|   18XX
[IBIS ver]   4.1
[File name]   18xx.ibs
[File Rev]   1.0
[Date]   Apr 18, 2014
[Source]   Data created at Texas Instruments India
[Disclaimer]   This information is for modeling purpose only, and is not
   guaranteed. The information is subject to change without
   notice.
[Copyright] Texas Instruments
|   Component 18XX
[Component]   18XX
[Manufacturer]   Texas Instruments.
[Package]
| variable   typ   min   max
R_pkg   0.35113   0.0058816   1.09261
L_pkg   8.95381e-10   1.49981e-11   2.78616e-09
C_pkg   2.63203e-13   2.01059e-13   3.9667e-13
[Pin]  signal_name   model_name   R_pin   L_pin   C_pin
A1   VSS_WL   NC   0   0   0
A2   RF_IN1_A_WL   NC   0   0   0
A3   VDD_OUT_VCO_WL   NC   0   0   0
A4   RF_IN2_A_WL   NC   0   0   0
A5   VSS_ANT_BG_WL   NC   0   0   0
A6   VDD_IN_PA_BG_WL   NC   0   0   0
A7   RF_IO1_BG_WL   NC   0   0   0
A8   VSS_RF_BT   NC   0   0   0
A9   RF_IO_BT   NC   0   0   0
A10  VSS_DCO_BT   NC   0   0   0
A11  VPP   NC   0   0   0
B1   RF_OUT_A_WL   NC   0   0   0
B2   VSS_PA_A_WL   NC   0   0   0
B3   VSS_VCO_WL   NC   0   0   0
B4   DEPOP   NC   0   0   0
B5   VDD_OUT_RF_WL   NC   0   0   0
B6   VSS_RF_WL   NC   0   0   0
B7   VSS_RF_WL   NC   0   0   0
B8   VDD_OUT_PPA_IF_BT   NC   0   0   0
B9   VDD_OUT_RF_BT   NC   0   0   0
B10  VDD_OUT_DCO_BT   NC   0   0   0
B11  FUNC2_BT   BQ18PROGHHVHYFBPB_IUANV_6LM   0.107178   2.73303e-10   2.19292e-13
C1   VSS_ANT_WL   NC   0   0   0
C2   VDD_IN_PA_WL   NC   0   0   0
C3   LDO_IN_WL   NC   0   0   0
C4   VDD_OUT_ANA_WL   NC   0   0   0
C5   VSS_ANA_WL   NC   0   0   0
C6   PDET_IN_FEM_TESTM_WL   OQ18120COMPFZPD_IUAJH_6LM   1.09261   2.78616e-09   3.9667e-13
C7   PABIAS_OUT_FEM_TESTP_WL   NC   0   0   0
C8   VDD_OUT_PA_BT   NC   0   0   0
C9   LDO_IN_PA_BT   NC   0   0   0
C10  LDO_IN_BT   NC   0   0   0
C11  VIO_IN   NC   0   0   0
D1   RF_IO2_BG_WL   NC   0   0   0
D2   VSS_PA_BG_WL   NC   0   0   0
D3   DC2DC_REQ_OUT   BQ18PROGHHVHYFBPB_IUANH_6LM   0.419876   1.07068e-09   2.75578e-13
D4   VSS_CLK   NC   0   0   0
D5   VSS   NC   0   0   0
D6   RF_SW_WL   NC   0   0   0
D7   VDD_DIG   NC   0   0   0
D8   SDIO_CMD_WL   BQ18PROGHHVHYFBPB_IUANH_6LM   0.529399   1.34997e-09   2.95292e-13
D9   VSS   NC   0   0   0
D10  SDIO_D3_WL   BQ18PROGHHVHYFBPB_IUANH_6LM   0.225237   5.74355e-10   2.40543e-13
D11  SDIO_D2_WL   BQ18PROGHHVHYFBPB_IUANH_6LM   0.0531736   1.35593e-10   2.09571e-13
E1   WL_EN   IQ18HHVHYSINK_IUAJH_6LM   0.0467988   1.19337e-10   2.08424e-13
E2   BT_EN   IQ18HHVHYSINK_IUAJH_6LM   0.20561   5.24306e-10   2.3701e-13
E3   IRQ_WL   BQ18PROGHHVHYFBPB_IUANH_6LM   0.357414   9.11405e-10   2.64334e-13
E4   CLK_IN_P   NC   0   0   0
E5   CLK_IN_M   NC   0   0   0
E6   RF_SW_BT   NC   0   0   0
E7   HCI_RX_BT   BQ18PROGHHVHYFBPB_IUANH_6LM   0.614975   1.56819e-09   3.10695e-13
E8   FUNC1_BT   BQ18PROGHHVHYFBPB_IUANV_6LM   0.491606   1.2536e-09   2.88489e-13
E9   SDIO_D1_WL   BQ18PROGHHVHYFBPB_IUANH_6LM   0.34553   8.81102e-10   2.62195e-13
E10  SDIO_D0_WL   BQ18PROGHHVHYFBPB_IUANH_6LM   0.210326   5.36332e-10   2.37859e-13
E11  SDIO_CLK_WL   BQ18PROGHHVHYFBPB_IUANH_6LM   0.0593028   1.51222e-10   2.10675e-13
F1   TX_SW_FEM_WL   BQ18SMART1HYFBPB_IUAJH_6LM   0.0551497   1.40632e-10   2.09927e-13
F2   PA_EN_FEM_WL   BQ18SMART1HYFBPB_IUAJH_6LM   0.20123   5.13136e-10   2.36221e-13
F3   RX_SW_FEM_WL   BQ18SMART1HYFBPB_IUAJH_6LM   0.351615   8.96619e-10   2.63291e-13
F4   RF_SW_1P8V_WL   BQ18SMART1HYFBPB_IUAJH_6LM   0.49319   1.25763e-09   2.88774e-13
F5   VDD_DIG   NC   0   0   0
F6   HCI_CTS_BT   BQ18PROGHHVHYFBPB_IUANH_6LM   0.751778   1.91703e-09   3.3532e-13
F7   HCI_TX_BT   BQ18PROGHHVHYFBPB_IUANH_6LM   0.621592   1.58506e-09   3.11886e-13
F8   I2S_FSYNC_FM   BQ18PROGHHVHYFBPB_IUANV_6LM   0.484723   1.23604e-09   2.8725e-13
F9   I2S_IN_FM   BQ18PROGHHVHYFBPB_IUANV_6LM   0.353731   9.02013e-10   2.63672e-13
F10  I2S_OUT_FM   BQ18PROGHHVHYFBPB_IUANH_6LM   0.219834   5.60576e-10   2.3957e-13
F11  I2S_CLK_FM   BQ18PROGHHVHYFBPB_IUANH_6LM   0.0540117   1.3773e-10   2.09722e-13
G1   VIO1_IN   NC   0   0   0
G2   UART_DBG_BT   BQ18PROGHHVHYFBPB_IUANH_6LM   0.211895   5.40333e-10   2.38141e-13
G3   RF_SW_1P8V_BT   BQ18SMART1HYFBPB_IUAJH_6LM   0.342157   8.725e-10   2.61588e-13
G4   UART_DBG_WL   BQ18PROGHHVHYFBPB_IUANH_6LM   0.485075   1.23694e-09   2.87313e-13
G5   COEX_MWS_UART_RX   BQ18SMART1HYFBPB_IUAJH_6LM   0.973323   2.48197e-09   3.75198e-13
G6   HCI_RTS_BT   BQ18PROGHHVHYFBPB_IUANH_6LM   0.852295   2.17335e-09   3.53413e-13
G7   COEX_MWS_UART_TX   BQ18SMART1HYFBPB_IUAJH_6LM   0.62343   1.58975e-09   3.12217e-13
G8   COEX_MWS_PRE_TX   BQ18SMART1HYFBPB_IUAJH_6LM   0.539399   1.37547e-09   2.97092e-13
G9   AUD_IN_BT   BQOMAPSLIMBUSFBPB_SSBHV_6LM   0.364435   9.29309e-10   2.65598e-13
G10  AUD_OUT_BT   OQ18120COMPFZPD_IUAJV_6LM   0.210935   5.37885e-10   2.37968e-13
G11  AUD_CLK_BT   BQ18PROGHHVHYFBPB_IUANV_6LM   0.0546034   1.39239e-10   2.09829e-13
H1   GPIO1   BQ18PROGHHVHYFBPB_IUANH_6LM   0.0429032   1.09403e-10   2.07723e-13
H2   GPIO2   BQ18PROGHHVHYFBPB_IUANH_6LM   0.210882   5.3775e-10   2.37959e-13
H3   GPIO4   BQ18PROGHHVHYFBPB_IUANH_6LM   0.344493   8.78457e-10   2.62009e-13
H4   VSS   NC   0   0   0
H5   I2C_CLK_NFC   BQOMAPI2CHYFBPBRES_SSBHH_6LM  0.0293107   7.47424e-11   2.05276e-13
H6   I2C_DATA_NFC   BQOMAPI2CHYFBPBRES_SSBHH_6LM  0.315157   8.0365e-10   2.56728e-13
H7   COEX_MWS_FRAME_SYNC   BQ18SMART1HYFBPB_IUAJV_6LM   0.753924   1.92251e-09   3.35706e-13
H8   RTC_CLK   IQ18HHVHYPDFS_IUAJV_6LM   0.679359   1.73237e-09   3.22285e-13
H9   VDD_DIG   NC   0   0   0
H10  VIO_IN   NC   0   0   0
H11  AUD_FSYNC_BT   BQOMAPSLIMBUSFBPB_SSBHV_6LM   0.0548647   1.39905e-10   2.09876e-13
J1   VBAT_IN_PA_DC2DC   NC   0   0   0
J2   PA_DC2DC_OUT   NC   0   0   0
J3   FB_IN_PA_DC2DC   NC   0   0   0
J4   SE_CLK_WIO_NFC   NC   0.0058816   1.49981e-11   2.01059e-13
J5   VSS_ANA_NFC   NC   0   0   0
J6   VSS_PLL_NFC   NC   0   0   0
J7   SWP_IO_NFC   NC   0   0   0
J8   AUD_OUT_L_FM   OQ18120COMPFZPD_IUAJV_6LM   0.500078   1.2752e-09   2.90014e-13
J9   LDO_IN_FM   NC   0   0   0
J10  DC2DC_REQ_MODE   BQ18PROGHHVHYFBPB_IUANH_6LM   0.265172   6.76188e-10   2.47731e-13
J11  VSS   NC   0   0   0
K1   VSS_PA_DC2DC   NC   0   0   0
K2   DIG_DC2DC_OUT   NC   0   0   0
K3   VDD_RAM   NC   0   0   0
K4   SE_IO_WII_NFC   NC   0.150559   3.83924e-10   2.27101e-13
K5   VDD_OUT_PER_NFC   NC   0   0   0
K6   FPSU_OUT_NFC   NC   0   0   0
K7   VDD_SWP_IN_NFC   NC   0   0   0
K8   AUD_OUT_R_FM   OQ18120COMPFZPD_IUAJV_6LM   0.34883   8.89516e-10   2.62789e-13
K9   VSS_PA_SYNTH_FM   NC   0   0   0
K10  DEPOP   NC   0   0   0
K11  CLK_REQ_OUT   BQ18PROGHHVHYFBPB_IUANH_6LM   0.149382   3.80925e-10   2.26889e-13
L1   VBAT_IN_MAIN_DC2DC   NC   0   0   0
L2   MAIN_DC2DC_OUT   NC   0   0   0
L3   LDO_IN_DIG   NC   0   0   0
L4   VBAT_IN_NFC   NC   0   0   0
L5   READER_P_NFC   NC   0   0   0
L6   VSS_PA_NFC   NC   0   0   0
L7   VDD_SWP_OUT_NFC   NC   0   0   0
L8   VSS_AUD_FM   NC   0   0   0
L9   VSS_RF_FM   NC   0   0   0
L10  VDD_OUT_PA_FM   NC   0   0   0
L11  RF_OUT_P_FM   NC   0   0   0
M1   TEST_PM   NC   0   0   0
M2   VSS_MAIN_DC2DC   NC   0   0   0
M3   VSS_DIG_DC2DC   NC   0   0   0
M4   VDD_OUT_PA_NFC   NC   0   0   0
M5   READER_M_NFC   NC   0   0   0
M6   TAG_P_NFC   NC   0   0   0
M7   TAG_M_NFC   NC   0   0   0
M8   BGAP_FM   NC   0   0   0
M9   RF_IN_FM   NC   0   0   0
M10  RF_OUT_M_FM   NC   0   0   0
M11  VSS_PA_FM   NC   0   0   0
[Model Selector] BQ18PROGHHVHYFBPB_IUANH_6LM
BQ18PROGFBPB_H11_PUPDOFF_1P8  Cell operated at 1.8(nom)
|BQ18PROGFBPB_H11_PUPDOFF_1P8; BUFFER WITH PULLUP & PULLDOWN OFF WITH DS0=1
|, DS1=1
BQ18PROGHHVHYFBPB_H00_PD_1P8  Cell operated at 1.8(nom)
|BQ18PROGHHVHYFBPB_H00_PD_1P8; BUFFER WITH WEAK_PD_ON WITH DS0=0, DS1=0
BQ18PROGHHVHYFBPB_H11_PD_1P8  Cell operated at 1.8(nom)
|BQ18PROGHHVHYFBPB_H11_PD_1P8; BUFFER WITH WEAK_PD_ON WITH DS0=1, DS1=1
BQ18PROGFBPB_H01_PUPDOFF_1P8  Cell operated at 1.8(nom)
|BQ18PROGFBPB_H01_PUPDOFF_1P8; BUFFER WITH PULLUP & PULLDOWN OFF WITH DS0=1
|, DS1=0
BQ18PROGHHVHYFBPB_H00_PU_1P8  Cell operated at 1.8(nom)
|BQ18PROGHHVHYFBPB_H00_PU_1P8; BUFFER WITH WEAK_PU_ON WITH DS0=0, DS1=0
BQ18PROGFBPB_H10_PUPDOFF_1P8  Cell operated at 1.8(nom)
|BQ18PROGFBPB_H10_PUPDOFF_1P8; BUFFER WITH PULLUP & PULLDOWN OFF WITH DS0=0
|, DS1=1
BQ18PROGHHVHYFBPB_H11_PU_1P8  Cell operated at 1.8(nom)
|BQ18PROGHHVHYFBPB_H11_PU_1P8; BUFFER WITH WEAK_PU_ON WITH DS0=1, DS1=1
BQ18PROGHHVHYFBPB_H01_PD_1P8  Cell operated at 1.8(nom)
|BQ18PROGHHVHYFBPB_H01_PD_1P8; BUFFER WITH WEAK_PD_ON WITH DS0=1, DS1=0
BQ18PROGHHVHYFBPB_H10_PD_1P8  Cell operated at 1.8(nom)
|BQ18PROGHHVHYFBPB_H10_PD_1P8; BUFFER WITH WEAK_PD_ON WITH DS0=0, DS1=1
BQ18PROGFBPB_H00_PUPDOFF_1P8  Cell operated at 1.8(nom)
|BQ18PROGFBPB_H00_PUPDOFF_1P8; BUFFER WITH PULLUP & PULLDOWN OFF WITH DS0=0
|, DS1=0
BQ18PROGHHVHYFBPB_H01_PU_1P8  Cell operated at 1.8(nom)
|BQ18PROGHHVHYFBPB_H01_PU_1P8; BUFFER WITH WEAK_PU_ON WITH DS0=1, DS1=0
BQ18PROGHHVHYFBPB_H10_PU_1P8  Cell operated at 1.8(nom)
|BQ18PROGHHVHYFBPB_H10_PU_1P8; BUFFER WITH WEAK_PU_ON WITH DS0=0, DS1=1
[Model Selector] BQ18PROGHHVHYFBPB_IUANV_6LM
BQ18PROGFBPB_V11_PUPDOFF_1P8  Cell operated at 1.8(nom)
|BQ18PROGFBPB_V11_PUPDOFF_1P8; BUFFER WITH PULLUP & PULLDOWN OFF WITH DS0=1
|, DS1=1
BQ18PROGHHVHYFBPB_V00_PD_1P8  Cell operated at 1.8(nom)
|BQ18PROGHHVHYFBPB_V00_PD_1P8; BUFFER WITH WEAK_PD_ON WITH DS0=0, DS1=0
BQ18PROGHHVHYFBPB_V11_PD_1P8  Cell operated at 1.8(nom)
|BQ18PROGHHVHYFBPB_V11_PD_1P8; BUFFER WITH WEAK_PD_ON WITH DS0=1, DS1=1
BQ18PROGFBPB_V01_PUPDOFF_1P8  Cell operated at 1.8(nom)
|BQ18PROGFBPB_V01_PUPDOFF_1P8; BUFFER WITH PULLUP & PULLDOWN OFF WITH DS0=1
|, DS1=0
BQ18PROGHHVHYFBPB_V00_PU_1P8  Cell operated at 1.8(nom)
|BQ18PROGHHVHYFBPB_V00_PU_1P8; BUFFER WITH WEAK_PU_ON WITH DS0=0, DS1=0
BQ18PROGFBPB_V10_PUPDOFF_1P8  Cell operated at 1.8(nom)
|BQ18PROGFBPB_V10_PUPDOFF_1P8; BUFFER WITH PULLUP & PULLDOWN OFF WITH DS0=0
|, DS1=1
BQ18PROGHHVHYFBPB_V11_PU_1P8  Cell operated at 1.8(nom)
|BQ18PROGHHVHYFBPB_V11_PU_1P8; BUFFER WITH WEAK_PU_ON WITH DS0=1, DS1=1
BQ18PROGHHVHYFBPB_V01_PD_1P8  Cell operated at 1.8(nom)
|BQ18PROGHHVHYFBPB_V01_PD_1P8; BUFFER WITH WEAK_PD_ON WITH DS0=1, DS1=0
BQ18PROGHHVHYFBPB_V10_PD_1P8  Cell operated at 1.8(nom)
|BQ18PROGHHVHYFBPB_V10_PD_1P8; BUFFER WITH WEAK_PD_ON WITH DS0=0, DS1=1
BQ18PROGFBPB_V00_PUPDOFF_1P8  Cell operated at 1.8(nom)
|BQ18PROGFBPB_V00_PUPDOFF_1P8; BUFFER WITH PULLUP & PULLDOWN OFF WITH DS0=0
|, DS1=0
BQ18PROGHHVHYFBPB_V01_PU_1P8  Cell operated at 1.8(nom)
|BQ18PROGHHVHYFBPB_V01_PU_1P8; BUFFER WITH WEAK_PU_ON WITH DS0=1, DS1=0
BQ18PROGHHVHYFBPB_V10_PU_1P8  Cell operated at 1.8(nom)
|BQ18PROGHHVHYFBPB_V10_PU_1P8; BUFFER WITH WEAK_PU_ON WITH DS0=0, DS1=1
[Model Selector] BQ18SMART1HYFBPB_IUAJH_6LM
BQ18SMART1HYFBPB_HS00L01_PU1_1P8  Cell operated at 1.8(nom)
|BQ18SMART1HYFBPB_HS00L01_PU1_1P8; BUFFER WITH WEAK_PULLUP_ON FOR SC1&&SC0=
|00:LB1&&LB0=01
BQ18SMART1HYFBPB_HS01L11_PD1_1P8  Cell operated at 1.8(nom)
|BQ18SMART1HYFBPB_HS01L11_PD1_1P8; BUFFER WITH WEAK_PULLDOWN_ON FOR SC1&&SC
|0=01:LB1&&LB0=11
BQ18SMART1HYFBPB_HS01L10_PD1_1P8  Cell operated at 1.8(nom)
|BQ18SMART1HYFBPB_HS01L10_PD1_1P8; BUFFER WITH WEAK_PULLDOWN_ON FOR SC1&&SC
|0=01:LB1&&LB0=10
BQ18SMART1HYFBPB_HS11L11_PU1_1P8  Cell operated at 1.8(nom)
|BQ18SMART1HYFBPB_HS11L11_PU1_1P8; BUFFER WITH WEAK_PULLUP_ON FOR SC1&&SC0=
|11:LB1&&LB0=11
BQ18SMART1HYFBPB_HS00L11_PD1_1P8  Cell operated at 1.8(nom)
|BQ18SMART1HYFBPB_HS00L11_PD1_1P8; BUFFER WITH WEAK_PULLDOWN_ON FOR SC1&&SC
|0=00:LB1&&LB0=11
BQ18SMART1HYFBPB_HS11L10_PUPD0_1P8  Cell operated at 1.8(nom)
|BQ18SMART1HYFBPB_HS11L10_PUPD0_1P8; BUFFER WITH PULLUP AND PULLDOWN OFF FO
|R SC0&&SC1=11:LB0&&LB1=10
BQ18SMART1HYFBPB_HS10L11_PU1_1P8  Cell operated at 1.8(nom)
|BQ18SMART1HYFBPB_HS10L11_PU1_1P8; BUFFER WITH WEAK_PULLUP_ON FOR SC1&&SC0=
|10:LB1&&LB0=11
BQ18SMART1HYFBPB_HS00L10_PD1_1P8  Cell operated at 1.8(nom)
|BQ18SMART1HYFBPB_HS00L10_PD1_1P8; BUFFER WITH WEAK_PULLDOWN_ON FOR SC1&&SC
|0=00:LB1&&LB0=10
BQ18SMART1HYFBPB_HS10L10_PUPD0_1P8  Cell operated at 1.8(nom)
|BQ18SMART1HYFBPB_HS10L10_PUPD0_1P8; BUFFER WITH PULLUP AND PULLDOWN OFF FO
|R SC1&&SC0=10:LB1&&LB0=10
BQ18SMART1HYFBPB_HS10L10_PU1_1P8  Cell operated at 1.8(nom)
|BQ18SMART1HYFBPB_HS10L10_PU1_1P8; BUFFER WITH WEAK_PULLUP_ON FOR SC1&&SC0=
|10:LB1&&LB0=10
BQ18SMART1HYFBPB_HS11L00_PUPD0_1P8  Cell operated at 1.8(nom)
|BQ18SMART1HYFBPB_HS11L00_PUPD0_1P8; BUFFER WITH PULLUP AND PULLDOWN OFF FO
|R SC0&&SC1=11:LB0&&LB1=00
BQ18SMART1HYFBPB_HS00L01_PD1_1P8  Cell operated at 1.8(nom)
|BQ18SMART1HYFBPB_HS00L01_PD1_1P8; BUFFER WITH WEAK_PULLDOWN_ON FOR SC1&&SC
|0=00:LB1&&LB0=01
BQ18SMART1HYFBPB_HS10L01_PUPD0_1P8  Cell operated at 1.8(nom)
|BQ18SMART1HYFBPB_HS10L01_PUPD0_1P8; BUFFER WITH PULLUP AND PULLDOWN OFF FO
|R SC1&&SC0=10:LB1&&LB0=01
BQ18SMART1HYFBPB_HS10L00_PUPD0_1P8  Cell operated at 1.8(nom)
|BQ18SMART1HYFBPB_HS10L00_PUPD0_1P8; BUFFER WITH PULLUP AND PULLDOWN OFF FO
|R SC1&&SC0=10:LB0&&LB1=00
BQ18SMART1HYFBPB_HS11L11_PD1_1P8  Cell operated at 1.8(nom)
|BQ18SMART1HYFBPB_HS11L11_PD1_1P8; BUFFER WITH WEAK_PULLDOWN_ON FOR SC1&&SC
|0=11:LB1&&LB0=11
BQ18SMART1HYFBPB_HS01L11_PU1_1P8  Cell operated at 1.8(nom)
|BQ18SMART1HYFBPB_HS01L11_PU1_1P8; BUFFER WITH WEAK_PULLUP_ON FOR SC1&&SC0=
|01:LB1&&LB0=11
BQ18SMART1HYFBPB_HS01L10_PUPD0_1P8  Cell operated at 1.8(nom)
|BQ18SMART1HYFBPB_HS01L10_PUPD0_1P8; BUFFER WITH PULLUP AND PULLDOWN OFF FO
|R SC1&&SC0=01:LB1&&LB0=10
BQ18SMART1HYFBPB_HS01L10_PU1_1P8  Cell operated at 1.8(nom)
|BQ18SMART1HYFBPB_HS01L10_PU1_1P8; BUFFER WITH WEAK_PULLUP_ON FOR SC1&&SC0=
|01:LB1&&LB0=10
BQ18SMART1HYFBPB_HS10L01_PD1_1P8  Cell operated at 1.8(nom)
|BQ18SMART1HYFBPB_HS10L01_PD1_1P8; BUFFER WITH WEAK_PULLDOWN_ON FOR SC1&&SC
|0=10:LB1&&LB0=01
BQ18SMART1HYFBPB_HS01L01_PUPD0_1P8  Cell operated at 1.8(nom)
|BQ18SMART1HYFBPB_HS01L01_PUPD0_1P8; BUFFER WITH PULLUP AND PULLDOWN OFF FO
|R SC1&&SC0=01:LB1&&LB0=01
BQ18SMART1HYFBPB_HS01L00_PUPD0_1P8  Cell operated at 1.8(nom)
|BQ18SMART1HYFBPB_HS01L00_PUPD0_1P8; BUFFER WITH PULLUP AND PULLDOWN OFF FO
|R SC1&&SC0=01:LB0&&LB1=00
BQ18SMART1HYFBPB_HS10L00_PD1_1P8  Cell operated at 1.8(nom)
|BQ18SMART1HYFBPB_HS10L00_PD1_1P8; BUFFER WITH WEAK_PULLDOWN_ON FOR SC1&&SC
|0=10:LB1&&LB0=00
BQ18SMART1HYFBPB_HS00L01_PUPD0_1P8  Cell operated at 1.8(nom)
|BQ18SMART1HYFBPB_HS00L01_PUPD0_1P8; BUFFER WITH PULLUP AND PULLDOWN OFF FO
|R SC1&&SC0=00:LB1&&LB0=01
BQ18SMART1HYFBPB_HS00L00_PUPD0_1P8  Cell operated at 1.8(nom)
|BQ18SMART1HYFBPB_HS00L00_PUPD0_1P8; BUFFER WITH PULLUP AND PULLDOWN OFF FO
|R SC0&&SC1=00:LB0&&LB1=00
BQ18SMART1HYFBPB_HS00L00_PU1_1P8  Cell operated at 1.8(nom)
|BQ18SMART1HYFBPB_HS00L00_PU1_1P8; BUFFER WITH WEAK_PULLUP_ON FOR SC1&&SC0=
|00:LB1&&LB0=00
BQ18SMART1HYFBPB_HS11L10_PU1_1P8  Cell operated at 1.8(nom)
|BQ18SMART1HYFBPB_HS11L10_PU1_1P8; BUFFER WITH WEAK_PULLUP_ON FOR SC1&&SC0=
|11:LB1&&LB0=10
BQ18SMART1HYFBPB_HS11L11_PUPD0_1P8  Cell operated at 1.8(nom)
|BQ18SMART1HYFBPB_HS11L11_PUPD0_1P8; BUFFER WITH PULLUP AND PULLDOWN OFF FO
|R SC0&&SC1=11:LB0&&LB1=11
BQ18SMART1HYFBPB_HS10L11_PUPD0_1P8  Cell operated at 1.8(nom)
|BQ18SMART1HYFBPB_HS10L11_PUPD0_1P8; BUFFER WITH PULLUP AND PULLDOWN OFF FO
|R SC1&&SC0=10:LB1&&LB0=11
BQ18SMART1HYFBPB_HS01L01_PD1_1P8  Cell operated at 1.8(nom)
|BQ18SMART1HYFBPB_HS01L01_PD1_1P8; BUFFER WITH WEAK_PULLDOWN_ON FOR SC1&&SC
|0=01:LB1&&LB0=01
BQ18SMART1HYFBPB_HS11L01_PU1_1P8  Cell operated at 1.8(nom)
|BQ18SMART1HYFBPB_HS11L01_PU1_1P8; BUFFER WITH WEAK_PULLUP_ON FOR SC1&&SC0=
|11:LB1&&LB0=01
BQ18SMART1HYFBPB_HS11L01_PUPD0_1P8  Cell operated at 1.8(nom)
|BQ18SMART1HYFBPB_HS11L01_PUPD0_1P8; BUFFER WITH PULLUP AND PULLDOWN OFF FO
|R SC0&&SC1=11:LB0&&LB1=01
BQ18SMART1HYFBPB_HS01L00_PD1_1P8  Cell operated at 1.8(nom)
|BQ18SMART1HYFBPB_HS01L00_PD1_1P8; BUFFER WITH WEAK_PULLDOWN_ON FOR SC1&&SC
|0=01:LB1&&LB0=00
BQ18SMART1HYFBPB_HS11L00_PU1_1P8  Cell operated at 1.8(nom)
|BQ18SMART1HYFBPB_HS11L00_PU1_1P8; BUFFER WITH WEAK_PULLUP_ON FOR SC1&&SC0=
|11:LB1&&LB0=00
BQ18SMART1HYFBPB_HS10L01_PU1_1P8  Cell operated at 1.8(nom)
|BQ18SMART1HYFBPB_HS10L01_PU1_1P8; BUFFER WITH WEAK_PULLUP_ON FOR SC1&&SC0=
|10:LB1&&LB0=01
BQ18SMART1HYFBPB_HS00L00_PD1_1P8  Cell operated at 1.8(nom)
|BQ18SMART1HYFBPB_HS00L00_PD1_1P8; BUFFER WITH WEAK_PULLDOWN_ON FOR SC1&&SC
|0=00:LB1&&LB0=00
BQ18SMART1HYFBPB_HS10L00_PU1_1P8  Cell operated at 1.8(nom)
|BQ18SMART1HYFBPB_HS10L00_PU1_1P8; BUFFER WITH WEAK_PULLUP_ON FOR SC1&&SC0=
|10:LB1&&LB0=00
BQ18SMART1HYFBPB_HS11L10_PD1_1P8  Cell operated at 1.8(nom)
|BQ18SMART1HYFBPB_HS11L10_PD1_1P8; BUFFER WITH WEAK_PULLDOWN_ON FOR SC1&&SC
|0=11:LB1&&LB0=10
BQ18SMART1HYFBPB_HS10L11_PD1_1P8  Cell operated at 1.8(nom)
|BQ18SMART1HYFBPB_HS10L11_PD1_1P8; BUFFER WITH WEAK_PULLDOWN_ON FOR SC1&&SC
|0=10:LB1&&LB0=11
BQ18SMART1HYFBPB_HS01L11_PUPD0_1P8  Cell operated at 1.8(nom)
|BQ18SMART1HYFBPB_HS01L11_PUPD0_1P8; BUFFER WITH PULLUP AND PULLDOWN OFF FO
|R SC1&&SC0=01:LB1&&LB0=11
BQ18SMART1HYFBPB_HS10L10_PD1_1P8  Cell operated at 1.8(nom)
|BQ18SMART1HYFBPB_HS10L10_PD1_1P8; BUFFER WITH WEAK_PULLDOWN_ON FOR SC1&&SC
|0=10:LB1&&LB0=10
BQ18SMART1HYFBPB_HS11L01_PD1_1P8  Cell operated at 1.8(nom)
|BQ18SMART1HYFBPB_HS11L01_PD1_1P8; BUFFER WITH WEAK_PULLDOWN_ON FOR SC1&&SC
|0=11:LB1&&LB0=01
BQ18SMART1HYFBPB_HS00L11_PU1_1P8  Cell operated at 1.8(nom)
|BQ18SMART1HYFBPB_HS00L11_PU1_1P8; BUFFER WITH WEAK_PULLUP_ON FOR SC1&&SC0=
|00:LB1&&LB0=11
BQ18SMART1HYFBPB_HS00L11_PUPD0_1P8  Cell operated at 1.8(nom)
|BQ18SMART1HYFBPB_HS00L11_PUPD0_1P8; BUFFER WITH PULLUP AND PULLDOWN OFF FO
|R SC1&&SC0=00:LB1&&LB0=11
BQ18SMART1HYFBPB_HS11L00_PD1_1P8  Cell operated at 1.8(nom)
|BQ18SMART1HYFBPB_HS11L00_PD1_1P8; BUFFER WITH WEAK_PULLDOWN_ON FOR SC1&&SC
|0=11:LB1&&LB0=00
BQ18SMART1HYFBPB_HS00L10_PUPD0_1P8  Cell operated at 1.8(nom)
|BQ18SMART1HYFBPB_HS00L10_PUPD0_1P8; BUFFER WITH PULLUP AND PULLDOWN OFF FO
|R SC1&&SC0=00:LB1&&LB0=10
BQ18SMART1HYFBPB_HS01L01_PU1_1P8  Cell operated at 1.8(nom)
|BQ18SMART1HYFBPB_HS01L01_PU1_1P8; BUFFER WITH WEAK_PULLUP_ON FOR SC1&&SC0=
|01:LB1&&LB0=01
BQ18SMART1HYFBPB_HS00L10_PU1_1P8  Cell operated at 1.8(nom)
|BQ18SMART1HYFBPB_HS00L10_PU1_1P8; BUFFER WITH WEAK_PULLUP_ON FOR SC1&&SC0=
|00:LB1&&LB0=10
BQ18SMART1HYFBPB_HS01L00_PU1_1P8  Cell operated at 1.8(nom)
|BQ18SMART1HYFBPB_HS01L00_PU1_1P8; BUFFER WITH WEAK_PULLUP_ON FOR SC1&&SC0=
|01:LB1&&LB0=00
[Model Selector] BQ18SMART1HYFBPB_IUAJV_6LM
BQ18SMART1HYFBPB_VS00L01_PU1_1P8  Cell operated at 1.8(nom)
|BQ18SMART1HYFBPB_VS00L01_PU1_1P8; BUFFER WITH WEAK_PULLUP_ON FOR SC1&&SC0=
|00:LB1&&LB0=01
BQ18SMART1HYFBPB_VS01L11_PD1_1P8  Cell operated at 1.8(nom)
|BQ18SMART1HYFBPB_VS01L11_PD1_1P8; BUFFER WITH WEAK_PULLDOWN_ON FOR SC1&&SC
|0=01:LB1&&LB0=11
BQ18SMART1HYFBPB_VS01L10_PD1_1P8  Cell operated at 1.8(nom)
|BQ18SMART1HYFBPB_VS01L10_PD1_1P8; BUFFER WITH WEAK_PULLDOWN_ON FOR SC1&&SC
|0=01:LB1&&LB0=10
BQ18SMART1HYFBPB_VS11L11_PU1_1P8  Cell operated at 1.8(nom)
|BQ18SMART1HYFBPB_VS11L11_PU1_1P8; BUFFER WITH WEAK_PULLUP_ON FOR SC1&&SC0=
|11:LB1&&LB0=11
BQ18SMART1HYFBPB_VS00L11_PD1_1P8  Cell operated at 1.8(nom)
|BQ18SMART1HYFBPB_VS00L11_PD1_1P8; BUFFER WITH WEAK_PULLDOWN_ON FOR SC1&&SC
|0=00:LB1&&LB0=11
BQ18SMART1HYFBPB_VS11L10_PUPD0_1P8  Cell operated at 1.8(nom)
|BQ18SMART1HYFBPB_VS11L10_PUPD0_1P8; BUFFER WITH PULLUP AND PULLDOWN OFF FO
|R SC0&&SC1=11:LB0&&LB1=10
BQ18SMART1HYFBPB_VS10L11_PU1_1P8  Cell operated at 1.8(nom)
|BQ18SMART1HYFBPB_VS10L11_PU1_1P8; BUFFER WITH WEAK_PULLUP_ON FOR SC1&&SC0=
|10:LB1&&LB0=11
BQ18SMART1HYFBPB_VS00L10_PD1_1P8  Cell operated at 1.8(nom)
|BQ18SMART1HYFBPB_VS00L10_PD1_1P8; BUFFER WITH WEAK_PULLDOWN_ON FOR SC1&&SC
|0=00:LB1&&LB0=10
BQ18SMART1HYFBPB_VS10L10_PUPD0_1P8  Cell operated at 1.8(nom)
|BQ18SMART1HYFBPB_VS10L10_PUPD0_1P8; BUFFER WITH PULLUP AND PULLDOWN OFF FO
|R SC1&&SC0=10:LB1&&LB0=10
BQ18SMART1HYFBPB_VS10L10_PU1_1P8  Cell operated at 1.8(nom)
|BQ18SMART1HYFBPB_VS10L10_PU1_1P8; BUFFER WITH WEAK_PULLUP_ON FOR SC1&&SC0=
|10:LB1&&LB0=10
BQ18SMART1HYFBPB_VS11L00_PUPD0_1P8  Cell operated at 1.8(nom)
|BQ18SMART1HYFBPB_VS11L00_PUPD0_1P8; BUFFER WITH PULLUP AND PULLDOWN OFF FO
|R SC0&&SC1=11:LB0&&LB1=00
BQ18SMART1HYFBPB_VS00L01_PD1_1P8  Cell operated at 1.8(nom)
|BQ18SMART1HYFBPB_VS00L01_PD1_1P8; BUFFER WITH WEAK_PULLDOWN_ON FOR SC1&&SC
|0=00:LB1&&LB0=01
BQ18SMART1HYFBPB_VS10L01_PUPD0_1P8  Cell operated at 1.8(nom)
|BQ18SMART1HYFBPB_VS10L01_PUPD0_1P8; BUFFER WITH PULLUP AND PULLDOWN OFF FO
|R SC1&&SC0=10:LB1&&LB0=01
BQ18SMART1HYFBPB_VS10L00_PUPD0_1P8  Cell operated at 1.8(nom)
|BQ18SMART1HYFBPB_VS10L00_PUPD0_1P8; BUFFER WITH PULLUP AND PULLDOWN OFF FO
|R SC1&&SC0=10:LB0&&LB1=00
BQ18SMART1HYFBPB_VS11L11_PD1_1P8  Cell operated at 1.8(nom)
|BQ18SMART1HYFBPB_VS11L11_PD1_1P8; BUFFER WITH WEAK_PULLDOWN_ON FOR SC1&&SC
|0=11:LB1&&LB0=11
BQ18SMART1HYFBPB_VS01L11_PU1_1P8  Cell operated at 1.8(nom)
|BQ18SMART1HYFBPB_VS01L11_PU1_1P8; BUFFER WITH WEAK_PULLUP_ON FOR SC1&&SC0=
|01:LB1&&LB0=11
BQ18SMART1HYFBPB_VS01L10_PUPD0_1P8  Cell operated at 1.8(nom)
|BQ18SMART1HYFBPB_VS01L10_PUPD0_1P8; BUFFER WITH PULLUP AND PULLDOWN OFF FO
|R SC1&&SC0=01:LB1&&LB0=10
BQ18SMART1HYFBPB_VS01L10_PU1_1P8  Cell operated at 1.8(nom)
|BQ18SMART1HYFBPB_VS01L10_PU1_1P8; BUFFER WITH WEAK_PULLUP_ON FOR SC1&&SC0=
|01:LB1&&LB0=10
BQ18SMART1HYFBPB_VS10L01_PD1_1P8  Cell operated at 1.8(nom)
|BQ18SMART1HYFBPB_VS10L01_PD1_1P8; BUFFER WITH WEAK_PULLDOWN_ON FOR SC1&&SC
|0=10:LB1&&LB0=01
BQ18SMART1HYFBPB_VS01L01_PUPD0_1P8  Cell operated at 1.8(nom)
|BQ18SMART1HYFBPB_VS01L01_PUPD0_1P8; BUFFER WITH PULLUP AND PULLDOWN OFF FO
|R SC1&&SC0=01:LB1&&LB0=01
BQ18SMART1HYFBPB_VS01L00_PUPD0_1P8  Cell operated at 1.8(nom)
|BQ18SMART1HYFBPB_VS01L00_PUPD0_1P8; BUFFER WITH PULLUP AND PULLDOWN OFF FO
|R SC1&&SC0=01:LB0&&LB1=00
BQ18SMART1HYFBPB_VS10L00_PD1_1P8  Cell operated at 1.8(nom)
|BQ18SMART1HYFBPB_VS10L00_PD1_1P8; BUFFER WITH WEAK_PULLDOWN_ON FOR SC1&&SC
|0=10:LB1&&LB0=00
BQ18SMART1HYFBPB_VS00L01_PUPD0_1P8  Cell operated at 1.8(nom)
|BQ18SMART1HYFBPB_VS00L01_PUPD0_1P8; BUFFER WITH PULLUP AND PULLDOWN OFF FO
|R SC1&&SC0=00:LB1&&LB0=01
BQ18SMART1HYFBPB_VS00L00_PUPD0_1P8  Cell operated at 1.8(nom)
|BQ18SMART1HYFBPB_VS00L00_PUPD0_1P8; BUFFER WITH PULLUP AND PULLDOWN OFF FO
|R SC0&&SC1=00:LB0&&LB1=00
BQ18SMART1HYFBPB_VS00L00_PU1_1P8  Cell operated at 1.8(nom)
|BQ18SMART1HYFBPB_VS00L00_PU1_1P8; BUFFER WITH WEAK_PULLUP_ON FOR SC1&&SC0=
|00:LB1&&LB0=00
BQ18SMART1HYFBPB_VS11L10_PU1_1P8  Cell operated at 1.8(nom)
|BQ18SMART1HYFBPB_VS11L10_PU1_1P8; BUFFER WITH WEAK_PULLUP_ON FOR SC1&&SC0=
|11:LB1&&LB0=10
BQ18SMART1HYFBPB_VS11L11_PUPD0_1P8  Cell operated at 1.8(nom)
|BQ18SMART1HYFBPB_VS11L11_PUPD0_1P8; BUFFER WITH PULLUP AND PULLDOWN OFF FO
|R SC0&&SC1=11:LB0&&LB1=11
BQ18SMART1HYFBPB_VS10L11_PUPD0_1P8  Cell operated at 1.8(nom)
|BQ18SMART1HYFBPB_VS10L11_PUPD0_1P8; BUFFER WITH PULLUP AND PULLDOWN OFF FO
|R SC1&&SC0=10:LB1&&LB0=11
BQ18SMART1HYFBPB_VS01L01_PD1_1P8  Cell operated at 1.8(nom)
|BQ18SMART1HYFBPB_VS01L01_PD1_1P8; BUFFER WITH WEAK_PULLDOWN_ON FOR SC1&&SC
|0=01:LB1&&LB0=01
BQ18SMART1HYFBPB_VS11L01_PU1_1P8  Cell operated at 1.8(nom)
|BQ18SMART1HYFBPB_VS11L01_PU1_1P8; BUFFER WITH WEAK_PULLUP_ON FOR SC1&&SC0=
|11:LB1&&LB0=01
BQ18SMART1HYFBPB_VS11L01_PUPD0_1P8  Cell operated at 1.8(nom)
|BQ18SMART1HYFBPB_VS11L01_PUPD0_1P8; BUFFER WITH PULLUP AND PULLDOWN OFF FO
|R SC0&&SC1=11:LB0&&LB1=01
BQ18SMART1HYFBPB_VS01L00_PD1_1P8  Cell operated at 1.8(nom)
|BQ18SMART1HYFBPB_VS01L00_PD1_1P8; BUFFER WITH WEAK_PULLDOWN_ON FOR SC1&&SC
|0=01:LB1&&LB0=00
BQ18SMART1HYFBPB_VS11L00_PU1_1P8  Cell operated at 1.8(nom)
|BQ18SMART1HYFBPB_VS11L00_PU1_1P8; BUFFER WITH WEAK_PULLUP_ON FOR SC1&&SC0=
|11:LB1&&LB0=00
BQ18SMART1HYFBPB_VS10L01_PU1_1P8  Cell operated at 1.8(nom)
|BQ18SMART1HYFBPB_VS10L01_PU1_1P8; BUFFER WITH WEAK_PULLUP_ON FOR SC1&&SC0=
|10:LB1&&LB0=01
BQ18SMART1HYFBPB_VS00L00_PD1_1P8  Cell operated at 1.8(nom)
|BQ18SMART1HYFBPB_VS00L00_PD1_1P8; BUFFER WITH WEAK_PULLDOWN_ON FOR SC1&&SC
|0=00:LB1&&LB0=00
BQ18SMART1HYFBPB_VS10L00_PU1_1P8  Cell operated at 1.8(nom)
|BQ18SMART1HYFBPB_VS10L00_PU1_1P8; BUFFER WITH WEAK_PULLUP_ON FOR SC1&&SC0=
|10:LB1&&LB0=00
BQ18SMART1HYFBPB_VS11L10_PD1_1P8  Cell operated at 1.8(nom)
|BQ18SMART1HYFBPB_VS11L10_PD1_1P8; BUFFER WITH WEAK_PULLDOWN_ON FOR SC1&&SC
|0=11:LB1&&LB0=10
BQ18SMART1HYFBPB_VS10L11_PD1_1P8  Cell operated at 1.8(nom)
|BQ18SMART1HYFBPB_VS10L11_PD1_1P8; BUFFER WITH WEAK_PULLDOWN_ON FOR SC1&&SC
|0=10:LB1&&LB0=11
BQ18SMART1HYFBPB_VS01L11_PUPD0_1P8  Cell operated at 1.8(nom)
|BQ18SMART1HYFBPB_VS01L11_PUPD0_1P8; BUFFER WITH PULLUP AND PULLDOWN OFF FO
|R SC1&&SC0=01:LB1&&LB0=11
BQ18SMART1HYFBPB_VS10L10_PD1_1P8  Cell operated at 1.8(nom)
|BQ18SMART1HYFBPB_VS10L10_PD1_1P8; BUFFER WITH WEAK_PULLDOWN_ON FOR SC1&&SC
|0=10:LB1&&LB0=10
BQ18SMART1HYFBPB_VS11L01_PD1_1P8  Cell operated at 1.8(nom)
|BQ18SMART1HYFBPB_VS11L01_PD1_1P8; BUFFER WITH WEAK_PULLDOWN_ON FOR SC1&&SC
|0=11:LB1&&LB0=01
BQ18SMART1HYFBPB_VS00L11_PU1_1P8  Cell operated at 1.8(nom)
|BQ18SMART1HYFBPB_VS00L11_PU1_1P8; BUFFER WITH WEAK_PULLUP_ON FOR SC1&&SC0=
|00:LB1&&LB0=11
BQ18SMART1HYFBPB_VS00L11_PUPD0_1P8  Cell operated at 1.8(nom)
|BQ18SMART1HYFBPB_VS00L11_PUPD0_1P8; BUFFER WITH PULLUP AND PULLDOWN OFF FO
|R SC1&&SC0=00:LB1&&LB0=11
BQ18SMART1HYFBPB_VS11L00_PD1_1P8  Cell operated at 1.8(nom)
|BQ18SMART1HYFBPB_VS11L00_PD1_1P8; BUFFER WITH WEAK_PULLDOWN_ON FOR SC1&&SC
|0=11:LB1&&LB0=00
BQ18SMART1HYFBPB_VS00L10_PUPD0_1P8  Cell operated at 1.8(nom)
|BQ18SMART1HYFBPB_VS00L10_PUPD0_1P8; BUFFER WITH PULLUP AND PULLDOWN OFF FO
|R SC1&&SC0=00:LB1&&LB0=10
BQ18SMART1HYFBPB_VS01L01_PU1_1P8  Cell operated at 1.8(nom)
|BQ18SMART1HYFBPB_VS01L01_PU1_1P8; BUFFER WITH WEAK_PULLUP_ON FOR SC1&&SC0=
|01:LB1&&LB0=01
BQ18SMART1HYFBPB_VS00L10_PU1_1P8  Cell operated at 1.8(nom)
|BQ18SMART1HYFBPB_VS00L10_PU1_1P8; BUFFER WITH WEAK_PULLUP_ON FOR SC1&&SC0=
|00:LB1&&LB0=10
BQ18SMART1HYFBPB_VS01L00_PU1_1P8  Cell operated at 1.8(nom)
|BQ18SMART1HYFBPB_VS01L00_PU1_1P8; BUFFER WITH WEAK_PULLUP_ON FOR SC1&&SC0=
|01:LB1&&LB0=00
[Model Selector] BQOMAPI2CHYFBPBRES_SSBHH_6LM
BQOMAPI2CHYRESNPM_SLV_PON_11_1P8  Cell operated at 1.8(nom)
|BQOMAPI2CHYRESNPM_SLV_PON_11_1P8; BUFFER IN HIGH SPEED SLAVE MODE WITH INT
|ERNAL PULLUP ON FOR LB1:LB0=11 FOR PAD LOAD 50-80PF
BQOMAPI2CHYRESNPM_SLV_PON_01_1P8  Cell operated at 1.8(nom)
|BQOMAPI2CHYRESNPM_SLV_PON_01_1P8; BUFFER IN HIGH SPEED SLAVE MODE WITH INT
|ERNAL PULLUP ON FOR LB1:LB0=01 FOR PAD LOAD 12-25PF
PI2CHYRESNPM_STD_FAST_INT_PULL_ON_01_1P8  Cell operated at 1.8(nom)
|BQOMAPI2CHYRESNPM_STD_FAST_INT_PULL_ON_01_1P8; BUFFER IN I2C STD_FAST MODE
| WITH INTERNAL PULLUP ON FOR LOAD 12-25PF LB1:LB0=01
BQOMAPI2CHYRESNPM_SLV_PON_10_1P8  Cell operated at 1.8(nom)
|BQOMAPI2CHYRESNPM_SLV_PON_10_1P8; BUFFER IN HIGH SPEED SLAVE MODE WITH INT
|ERNAL PULLUP ON FOR LB1:LB0=10 FOR PAD LOAD 25-50PF
PI2CHYRESNPM_STD_FAST_INT_PULL_ON_10_1P8  Cell operated at 1.8(nom)
|BQOMAPI2CHYRESNPM_STD_FAST_INT_PULL_ON_10_1P8; BUFFER IN I2C STD_FAST MODE
| WITH INTERNAL PULLUP ON FOR LOAD 25-50PF LB1:LB0=10
BQOMAPI2CHYRESNPM_SLV_PON_00_1P8  Cell operated at 1.8(nom)
|BQOMAPI2CHYRESNPM_SLV_PON_00_1P8; BUFFER IN HIGH SPEED SLAVE MODE WITH INT
|ERNAL PULLUP ON FOR LB1:LB0=00 FOR PAD LOAD 5-12PF
BQOMAPI2CHYRESNPM_SLV_EXT_PULLUP_1P8  Cell operated at 1.8(nom)
|BQOMAPI2CHYRESNPM_SLV_EXT_PULLUP_1P8; BUFFER IN HIGH SPEED SLAVE MODE WITH
| EXT PULLUP
PI2CHYRESNPM_STD_FAST_EXT_PULLUP_RES_1P8  Cell operated at 1.8(nom)
|BQOMAPI2CHYRESNPM_STD_FAST_EXT_PULLUP_RES_1P8; BUFFER IN I2C STD_FAST MODE
| WITH EXT PULLUP RES
PI2CHYRESNPM_STD_FAST_INT_PULL_ON_00_1P8  Cell operated at 1.8(nom)
|BQOMAPI2CHYRESNPM_STD_FAST_INT_PULL_ON_00_1P8; BUFFER IN I2C STD_FAST MODE
| WITH INTERNAL PULLUP ON FOR LOAD 5-12PF LB1:LB0=00
BQOMAPI2CHYRESNPM_LVCMOS_1P8  Cell operated at 1.8(nom)
|BQOMAPI2CHYRESNPM_LVCMOS_1P8; BUFFER IN LVCMOS PUSHPULL MODE
BQOMAPI2CHYRESNPM_SLV_PON_11_1P2  Cell operated at 1.2(nom)
|BQOMAPI2CHYRESNPM_SLV_PON_11_1P2; BUFFER IN HIGH SPEED SLAVE MODE WITH INT
|ERNAL PULLUP ON FOR LB1:LB0=11 FOR PAD LOAD 50-80PF
BQOMAPI2CHYRESNPM_SLV_PON_01_1P2  Cell operated at 1.2(nom)
|BQOMAPI2CHYRESNPM_SLV_PON_01_1P2; BUFFER IN HIGH SPEED SLAVE MODE WITH INT
|ERNAL PULLUP ON FOR LB1:LB0=01 FOR PAD LOAD 12-25PF
PI2CHYRESNPM_STD_FAST_INT_PULL_ON_01_1P2  Cell operated at 1.2(nom)
|BQOMAPI2CHYRESNPM_STD_FAST_INT_PULL_ON_01_1P2; BUFFER IN I2C STD_FAST MODE
| WITH INTERNAL PULLUP ON FOR LOAD 12-25PF LB1:LB0=01
BQOMAPI2CHYRESNPM_SLV_PON_10_1P2  Cell operated at 1.2(nom)
|BQOMAPI2CHYRESNPM_SLV_PON_10_1P2; BUFFER IN HIGH SPEED SLAVE MODE WITH INT
|ERNAL PULLUP ON FOR LB1:LB0=10 FOR PAD LOAD 25-50PF
PI2CHYRESNPM_STD_FAST_INT_PULL_ON_10_1P2  Cell operated at 1.2(nom)
|BQOMAPI2CHYRESNPM_STD_FAST_INT_PULL_ON_10_1P2; BUFFER IN I2C STD_FAST MODE
| WITH INTERNAL PULLUP ON FOR LOAD 25-50PF LB1:LB0=10
BQOMAPI2CHYRESNPM_SLV_PON_00_1P2  Cell operated at 1.2(nom)
|BQOMAPI2CHYRESNPM_SLV_PON_00_1P2; BUFFER IN HIGH SPEED SLAVE MODE WITH INT
|ERNAL PULLUP ON FOR LB1:LB0=00 FOR PAD LOAD 5-12PF
BQOMAPI2CHYRESNPM_SLV_EXT_PULLUP_1P2  Cell operated at 1.2(nom)
|BQOMAPI2CHYRESNPM_SLV_EXT_PULLUP_1P2; BUFFER IN HIGH SPEED SLAVE MODE WITH
| EXT PULLUP
PI2CHYRESNPM_STD_FAST_EXT_PULLUP_RES_1P2  Cell operated at 1.2(nom)
|BQOMAPI2CHYRESNPM_STD_FAST_EXT_PULLUP_RES_1P2; BUFFER IN I2C STD_FAST MODE
| WITH EXT PULLUP RES
PI2CHYRESNPM_STD_FAST_INT_PULL_ON_00_1P2  Cell operated at 1.2(nom)
|BQOMAPI2CHYRESNPM_STD_FAST_INT_PULL_ON_00_1P2; BUFFER IN I2C STD_FAST MODE
| WITH INTERNAL PULLUP ON FOR LOAD 5-12PF LB1:LB0=00
BQOMAPI2CHYRESNPM_LVCMOS_1P2  Cell operated at 1.2(nom)
|BQOMAPI2CHYRESNPM_LVCMOS_1P2; BUFFER IN LVCMOS PUSHPULL MODE
[Model Selector] BQOMAPSLIMBUSFBPB_SSBHV_6LM
BQOMAPSLIMBUS_V01_PUPD_1P8  Cell operated at 1.8(nom)
|BQOMAPSLIMBUS_V01_PUPD_1P8; BUFFER WITH PULLUP AND PULLDOWN OFF
BQOMAPSLIMBUS_V11_PU_1P8  Cell operated at 1.8(nom)
|BQOMAPSLIMBUS_V11_PU_1P8; BUFFER WITH WEAK_PULLUP_ON
BQOMAPSLIMBUS_V00_PD_1P8  Cell operated at 1.8(nom)
|BQOMAPSLIMBUS_V00_PD_1P8; BUFFER WITH WEAK_PULLDOWN_ON
BQOMAPSLIMBUS_V01_PD_1P8  Cell operated at 1.8(nom)
|BQOMAPSLIMBUS_V01_PD_1P8; BUFFER WITH WEAK_PULLDOWN_ON
BQOMAPSLIMBUS_V00_PU_1P8  Cell operated at 1.8(nom)
|BQOMAPSLIMBUS_V00_PU_1P8; BUFFER WITH WEAK_PULLUP_ON
BQOMAPSLIMBUS_V10_PUPD_1P8  Cell operated at 1.8(nom)
|BQOMAPSLIMBUS_V10_PUPD_1P8; BUFFER WITH PULLUP AND PULLDOWN OFF
BQOMAPSLIMBUS_V01_PU_1P8  Cell operated at 1.8(nom)
|BQOMAPSLIMBUS_V01_PU_1P8; BUFFER WITH WEAK_PULLUP_ON
BQOMAPSLIMBUS_V11_PUPD_1P8  Cell operated at 1.8(nom)
|BQOMAPSLIMBUS_V11_PUPD_1P8; BUFFER WITH PULLUP AND PULLDOWN OFF
BQOMAPSLIMBUS_V10_PD_1P8  Cell operated at 1.8(nom)
|BQOMAPSLIMBUS_V10_PD_1P8; BUFFER WITH WEAK_PULLDOWN_ON
BQOMAPSLIMBUS_V10_PU_1P8  Cell operated at 1.8(nom)
|BQOMAPSLIMBUS_V10_PU_1P8; BUFFER WITH WEAK_PULLUP_ON
BQOMAPSLIMBUS_V00_PUPD_1P8  Cell operated at 1.8(nom)
|BQOMAPSLIMBUS_V00_PUPD_1P8; BUFFER WITH PULLUP AND PULLDOWN OFF
BQOMAPSLIMBUS_V11_PD_1P8  Cell operated at 1.8(nom)
|BQOMAPSLIMBUS_V11_PD_1P8; BUFFER WITH WEAK_PULLDOWN_ON
[Model Selector] IQ18HHVHYPDFS_IUAJV_6LM
IQ18HHVHYPDF_V_PDOFF_1P8  Cell operated at 1.8(nom)
|IQ18HHVHYPDF_V_PDOFF_1P8; BUFFER IN NORMAL MODE WITH PULLDOWN OFF
IQ18HHVHYPDF_V_PD_ON_1P8  Cell operated at 1.8(nom)
|IQ18HHVHYPDF_V_PD_ON_1P8; BUFFER WITH WEAK_PULLDOWN_ON
[Model Selector] OQ18120COMPFZPD_IUAJH_6LM
OQ18120COMPF_H_PDOFF_1P8  Cell operated at 1.8(nom)
|OQ18120COMPF_H_PDOFF_1P8; BUFFER IN NORMAL MODE WITH PULLDOWN OFF
OQ18120COMPFZ_H_PDON_1P8  Cell operated at 1.8(nom)
|OQ18120COMPFZ_H_PDON_1P8; BUFFER WITH WEAK PULLDOWN ON
[Model Selector] OQ18120COMPFZPD_IUAJV_6LM
OQ18120COMPF_V_PDOFF_1P8  Cell operated at 1.8(nom)
|OQ18120COMPF_V_PDOFF_1P8; BUFFER IN NORMAL MODE WITH PULLDOWN OFF
OQ18120COMPFZ_V_PDON_1P8  Cell operated at 1.8(nom)
| Models and submodels in the file (159): BQ18PROGFBPB_H11_PUPDOFF_1P8 (I/O), BQ18PROGHHVHYFBPB_H00_PD_1P8 (I/O), BQ18PROGHHVHYFBPB_H11_PD_1P8 (I/O), BQ18PROGFBPB_H01_PUPDOFF_1P8 (I/O), BQ18PROGHHVHYFBPB_H00_PU_1P8 (I/O), BQ18PROGFBPB_H10_PUPDOFF_1P8 (I/O), BQ18PROGHHVHYFBPB_H11_PU_1P8 (I/O), BQ18PROGHHVHYFBPB_H01_PD_1P8 (I/O), BQ18PROGHHVHYFBPB_H10_PD_1P8 (I/O), BQ18PROGFBPB_H00_PUPDOFF_1P8 (I/O), BQ18PROGHHVHYFBPB_H01_PU_1P8 (I/O), BQ18PROGHHVHYFBPB_H10_PU_1P8 (I/O), BQ18PROGFBPB_V11_PUPDOFF_1P8 (I/O), BQ18PROGHHVHYFBPB_V00_PD_1P8 (I/O), BQ18PROGHHVHYFBPB_V11_PD_1P8 (I/O), BQ18PROGFBPB_V01_PUPDOFF_1P8 (I/O), BQ18PROGHHVHYFBPB_V00_PU_1P8 (I/O), BQ18PROGFBPB_V10_PUPDOFF_1P8 (I/O), BQ18PROGHHVHYFBPB_V11_PU_1P8 (I/O), BQ18PROGHHVHYFBPB_V01_PD_1P8 (I/O), BQ18PROGHHVHYFBPB_V10_PD_1P8 (I/O), BQ18PROGFBPB_V00_PUPDOFF_1P8 (I/O), BQ18PROGHHVHYFBPB_V01_PU_1P8 (I/O), BQ18PROGHHVHYFBPB_V10_PU_1P8 (I/O), BQ18SMART1HYFBPB_HS00L01_PU1_1P8 (I/O), BQ18SMART1HYFBPB_HS01L11_PD1_1P8 (I/O), BQ18SMART1HYFBPB_HS01L10_PD1_1P8 (I/O), BQ18SMART1HYFBPB_HS11L11_PU1_1P8 (I/O), BQ18SMART1HYFBPB_HS00L11_PD1_1P8 (I/O), BQ18SMART1HYFBPB_HS11L10_PUPD0_1P8 (I/O), BQ18SMART1HYFBPB_HS10L11_PU1_1P8 (I/O), BQ18SMART1HYFBPB_HS00L10_PD1_1P8 (I/O), BQ18SMART1HYFBPB_HS10L10_PUPD0_1P8 (I/O), BQ18SMART1HYFBPB_HS10L10_PU1_1P8 (I/O), BQ18SMART1HYFBPB_HS11L00_PUPD0_1P8 (I/O), BQ18SMART1HYFBPB_HS00L01_PD1_1P8 (I/O), BQ18SMART1HYFBPB_HS10L01_PUPD0_1P8 (I/O), BQ18SMART1HYFBPB_HS10L00_PUPD0_1P8 (I/O), BQ18SMART1HYFBPB_HS11L11_PD1_1P8 (I/O), BQ18SMART1HYFBPB_HS01L11_PU1_1P8 (I/O), BQ18SMART1HYFBPB_HS01L10_PUPD0_1P8 (I/O), BQ18SMART1HYFBPB_HS01L10_PU1_1P8 (I/O), BQ18SMART1HYFBPB_HS10L01_PD1_1P8 (I/O), BQ18SMART1HYFBPB_HS01L01_PUPD0_1P8 (I/O), BQ18SMART1HYFBPB_HS01L00_PUPD0_1P8 (I/O), BQ18SMART1HYFBPB_HS10L00_PD1_1P8 (I/O), BQ18SMART1HYFBPB_HS00L01_PUPD0_1P8 (I/O), BQ18SMART1HYFBPB_HS00L00_PUPD0_1P8 (I/O), BQ18SMART1HYFBPB_HS00L00_PU1_1P8 (I/O), BQ18SMART1HYFBPB_HS11L10_PU1_1P8 (I/O), BQ18SMART1HYFBPB_HS11L11_PUPD0_1P8 (I/O), BQ18SMART1HYFBPB_HS10L11_PUPD0_1P8 (I/O), BQ18SMART1HYFBPB_HS01L01_PD1_1P8 (I/O), BQ18SMART1HYFBPB_HS11L01_PU1_1P8 (I/O), BQ18SMART1HYFBPB_HS11L01_PUPD0_1P8 (I/O), BQ18SMART1HYFBPB_HS01L00_PD1_1P8 (I/O), BQ18SMART1HYFBPB_HS11L00_PU1_1P8 (I/O), BQ18SMART1HYFBPB_HS10L01_PU1_1P8 (I/O), BQ18SMART1HYFBPB_HS00L00_PD1_1P8 (I/O), BQ18SMART1HYFBPB_HS10L00_PU1_1P8 (I/O), BQ18SMART1HYFBPB_HS11L10_PD1_1P8 (I/O), BQ18SMART1HYFBPB_HS10L11_PD1_1P8 (I/O), BQ18SMART1HYFBPB_HS01L11_PUPD0_1P8 (I/O), BQ18SMART1HYFBPB_HS10L10_PD1_1P8 (I/O), BQ18SMART1HYFBPB_HS11L01_PD1_1P8 (I/O), BQ18SMART1HYFBPB_HS00L11_PU1_1P8 (I/O), BQ18SMART1HYFBPB_HS00L11_PUPD0_1P8 (I/O), BQ18SMART1HYFBPB_HS11L00_PD1_1P8 (I/O), BQ18SMART1HYFBPB_HS00L10_PUPD0_1P8 (I/O), BQ18SMART1HYFBPB_HS01L01_PU1_1P8 (I/O), BQ18SMART1HYFBPB_HS00L10_PU1_1P8 (I/O), BQ18SMART1HYFBPB_HS01L00_PU1_1P8 (I/O), BQ18SMART1HYFBPB_VS00L01_PU1_1P8 (I/O), BQ18SMART1HYFBPB_VS01L11_PD1_1P8 (I/O), BQ18SMART1HYFBPB_VS01L10_PD1_1P8 (I/O), BQ18SMART1HYFBPB_VS11L11_PU1_1P8 (I/O), BQ18SMART1HYFBPB_VS00L11_PD1_1P8 (I/O), BQ18SMART1HYFBPB_VS11L10_PUPD0_1P8 (I/O), BQ18SMART1HYFBPB_VS10L11_PU1_1P8 (I/O), BQ18SMART1HYFBPB_VS00L10_PD1_1P8 (I/O)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
